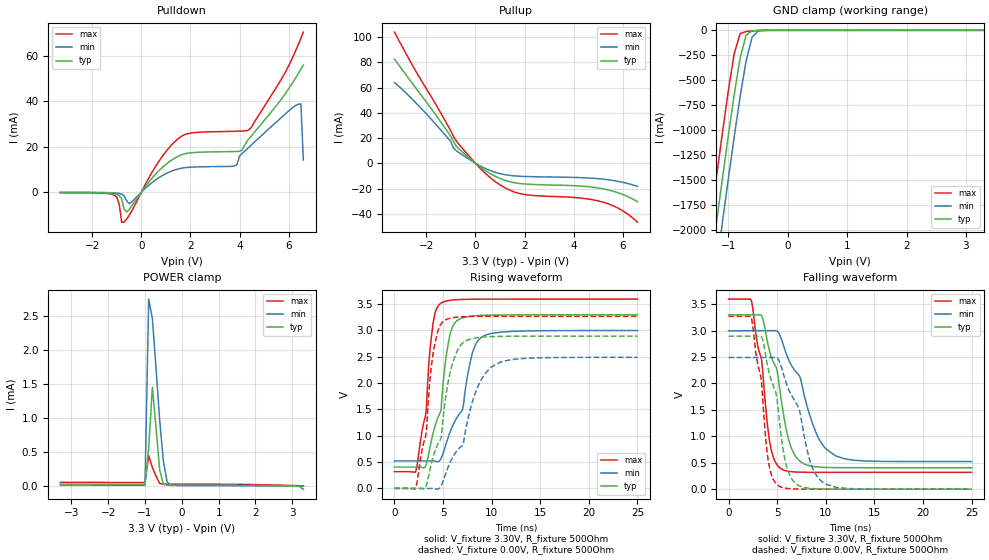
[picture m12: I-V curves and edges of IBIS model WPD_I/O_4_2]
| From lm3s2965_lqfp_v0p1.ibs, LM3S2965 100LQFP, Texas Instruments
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[Model]   WPD_I/O_4_2
Model_type   I/O
Vinl = 1.26
Vinh = 2.04
Vmeas = 1.65
| variable   typ   min   max
C_comp   9.739pF   9.739pF   9.739pF
[Model Spec]
Vinh+   1.91   1.78   2.04
Vinh-   1.90   1.76   2.03
Vinl+   1.40   1.27   1.54
Vinl-   1.39   1.26   1.53
| variable   typ   min   max
[Temperature Range]  25   85   -40
[Voltage Range]   3.3V   3.0V   3.6V
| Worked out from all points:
|   slope of the pulldown table from 0 to 0.495 V, typ, clamps not added: 71.6 ohm
|   slope of the pullup table from 0 to 0.495 V, typ, clamps not added: 71.6 ohm
|   GND clamp passes 1 mA (typ) near -0.48 V on its own axis
|   POWER clamp passes 1 mA (typ) near -0.72 V on its own axis
|   falling waveform, V_fixture 3.30V, R_fixture 500Ohm: 20-80 % time 2.03ns typ, 3.06ns min, 1.36ns max; typ from 3.3 V to 0.405 V
|   rising waveform, V_fixture 3.30V, R_fixture 500Ohm: 20-80 % time 1.62ns typ, 2.31ns min, 1.11ns max; typ from 0.405 V to 3.3 V
|   falling waveform, V_fixture 0.00V, R_fixture 500Ohm: 20-80 % time 1.75ns typ, 2.48ns min, 1.21ns max; typ from 2.89 V to 0 V
|   rising waveform, V_fixture 0.00V, R_fixture 500Ohm: 20-80 % time 1.94ns typ, 2.99ns min, 1.26ns max; typ from 0 V to 2.89 V
[Pulldown]
|  Voltage   I(typ)   I(min)   I(max)
-3.3V     -128.2uA   -72.79uA   -182.2uA
-1.1V     -636.2uA   -293.6uA   -1.283mA
-800mV    -2.996mA   -834.9uA   -13.19mA
-700mV    -7.354mA   -1.607mA   -13.15mA
-500mV    -7.623mA   -4.999mA   -10.32mA
700mV     9.301mA    6.299mA    13.36mA
1.6V      16.31mA    10.5mA     24.39mA
3.8V      17.93mA    11.6mA     26.84mA
4.4V      23.69mA    19.99mA    27.69mA
6.4V      52.4mA     38.79mA    65.21mA
6.5V      54.19mA    38.86mA    67.83mA
6.6V      55.99mA    14.2mA     70.53mA
[Pullup]
|  Voltage   I(typ)   I(min)   I(max)
-3.3V     82.55mA    63.93mA    103.9mA
-1.8V     43.23mA    34.85mA    52.65mA
-1V       21.12mA    17.2mA     25.41mA
-900mV    17.75mA    12.24mA    21.49mA
-800mV    14.04mA    10.31mA    18.31mA
100mV     -1.569mA   -1.126mA   -2.147mA
700mV     -9.236mA   -6.432mA   -12.93mA
1.3V      -14.09mA   -9.375mA   -20.39mA
1.9V      -16.21mA   -10.36mA   -24.42mA
5.2V      -20.25mA   -12.6mA    -30.84mA
5.9V      -24.02mA   -14.69mA   -36.54mA
6.6V      -30.45mA   -18.28mA   -46.68mA
[GND Clamp]
|  Voltage   I(typ)   I(min)   I(max)
-3.3V     -11.72A    -12.12A    -11.3A
-1.4V     -2.845A    -3.285A    -2.387A
-1.3V     -2.39A     -2.831A    -1.93A
-1.2V     -1.938A    -2.38A     -1.478A
-1.1V     -1.494A    -1.934A    -1.036A
-1V       -1.059A    -1.496A    -610.6mA
-900mV    -645mA     -1.069A    -232.9mA
-800mV    -277.1mA   -664.4mA   -31.59mA
-700mV    -48.56mA   -306.6mA   -12.1mA
-600mV    -5.561mA   -70.2mA    -6.281mA
-500mV    -1.172mA   -7.88mA    -2.176mA
3.3V      16.11uA    11.84uA    29.77uA
[POWER Clamp]
|  Voltage   I(typ)   I(min)   I(max)
-3.3V     31.42uA    17.14uA    57.54uA
-1V       30.25uA    16.5uA     55.43uA
-900mV    557.3uA    2.746mA    449.1uA
-800mV    1.452mA    2.463mA    276.5uA
-700mV    854.2uA    1.726mA    147.8uA
-600mV    235.9uA    958.2uA    41.01uA
-500mV    28.31uA    363.4uA    30.71uA
-400mV    16.41uA    67.09uA    29.83uA
-300mV    16.12uA    11.84uA    29.79uA
3.1V      2.408uA    -920.8nA   9.197uA
3.2V      1.227uA    -3.925uA   7.474uA
3.3V      -104.7pA   -42.65uA   5.692uA
[Ramp]
| variable   typ   min   max
dV/dt_f   1.73/2.03n   1.48/3.06n   1.97/1.36n
dV/dt_r   1.74/1.94n   1.49/2.99n   1.96/1.26n
R_load = 500Ohm
[Falling Waveform]
V_fixture = 3.30V
V_fixture_min = 3.00V
V_fixture_max = 3.60V
R_fixture = 500Ohm
|   Time   V(typ)   V(min)   V(max)
0s        3.297V     2.994V     3.595V
2.3ns     3.297V     2.997V     3.59V
3.4ns     3.283V     2.998V     2.441V
4.3ns     2.559V     2.998V     826.9mV
5.3ns     1.846V     2.901V     400mV
6.1ns     994.8mV    2.482V     339.4mV
6.9ns     620.2mV    2.226V     324.5mV
9.2ns     419.7mV    985.1mV    318.8mV
11ns      407.7mV    630.6mV    318.6mV
25ns      405.4mV    522.4mV    318.5mV
[Rising Waveform]
V_fixture = 3.30V
V_fixture_min = 3.00V
V_fixture_max = 3.60V
R_fixture = 500Ohm
|   Time   V(typ)   V(min)   V(max)
0s        405.4mV    522.4mV    318.5mV
2.2ns     405.4mV    522.4mV    327.6mV
3.2ns     420.5mV    522.4mV    1.383V
4ns       1.067V     522.1mV    3.164V
4.8ns     1.506V     570.5mV    3.521V
5.3ns     2.474V     838.3mV    3.558V
6ns       3.077V     1.194V     3.579V
7ns       3.239V     1.496V     3.59V
9ns       3.287V     2.875V     3.595V
25ns      3.298V     2.999V     3.597V
[Falling Waveform]
V_fixture = 0.00V
V_fixture_min = 0.00V
V_fixture_max = 0.00V
R_fixture = 500Ohm
|   Time   V(typ)   V(min)   V(max)
0s        2.893V     2.49V      3.27V
2.3ns     2.893V     2.491V     3.264V
3.4ns     2.877V     2.491V     2.005V
4.1ns     2.254V     2.491V     517.1mV
5.1ns     1.527V     2.462V     69.45mV
5.7ns     654.7mV    2.142V     23.49mV
6.4ns     225.2mV    1.803V     7.427mV
8.5ns     14.01mV    465.6mV    487.9uV
9.8ns     3.391mV    117.3mV    171.8uV
25ns      17.18uV    28.46uV    11.66uV
[Rising Waveform]
V_fixture = 0.00V
V_fixture_min = 0.00V
V_fixture_max = 0.00V
R_fixture = 500Ohm
|   Time   V(typ)   V(min)   V(max)
0s        186.9uV    3.8mV      10.44uV
2.2ns     29.21uV    789.5uV    11.85mV
3.3ns     69.38mV    374.1uV    1.1V
4ns       612.6mV    -32.31uV   2.589V
4.8ns     961.2mV    50.1mV     3.127V
5.1ns     1.486V     187.8mV    3.184V
6.7ns     2.693V     769.4mV    3.258V
8.4ns     2.859V     1.853V     3.267V
10ns      2.884V     2.312V     3.269V
25ns      2.893V     2.49V      3.269V
